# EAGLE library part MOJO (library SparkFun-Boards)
Mojo v3 FPGA Development Board Mechanical footprint with connectors for Mojo FPGA dev board. SparkFun Products: Mojo v3
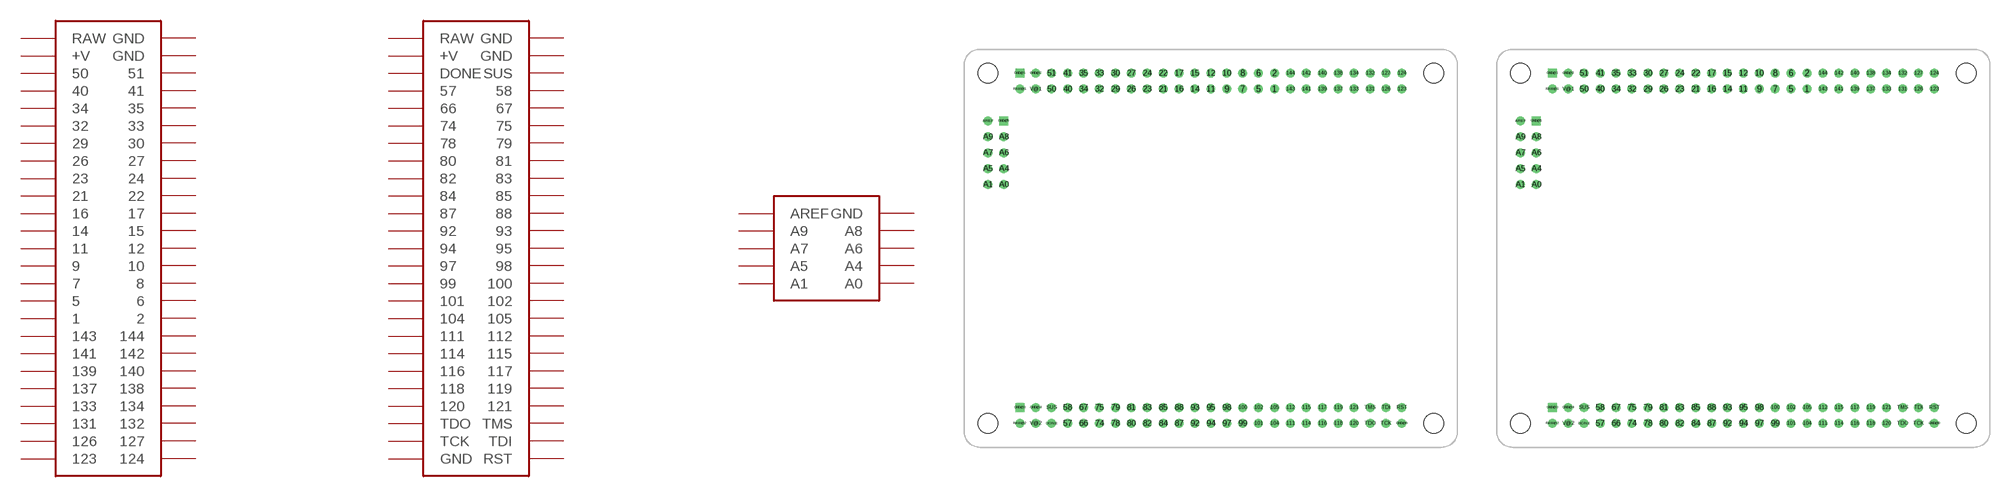
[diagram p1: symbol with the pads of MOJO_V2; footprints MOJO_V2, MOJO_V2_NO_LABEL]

Designator prefix B; gates G$1=MOJO_ANALOG_HEADER G$2=MOJO_HEADER_1 G$3=MOJO_HEADER_2

## MOJOV2  [MOJO_V2]
1  G$2:1
2  G$2:2
5  G$2:5
6  G$2:6
7  G$2:7
8  G$2:8
9  G$2:9
10  G$2:10
11  G$2:11
12  G$2:12
14  G$2:14
15  G$2:15
16  G$2:16
17  G$2:17
21  G$2:21
22  G$2:22
23  G$2:23
24  G$2:24
26  G$2:26
27  G$2:27
29  G$2:29
30  G$2:30
32  G$2:32
33  G$2:33
34  G$2:34
35  G$2:35
40  G$2:40
41  G$2:41
50  G$2:50
51  G$2:51
57  G$3:57
58  G$3:58
66  G$3:66
67  G$3:67
74  G$3:74
75  G$3:75
78  G$3:78
79  G$3:79
80  G$3:80
81  G$3:81
82  G$3:82
83  G$3:83
84  G$3:84
85  G$3:85
87  G$3:87
88  G$3:88
92  G$3:92
93  G$3:93
94  G$3:94
95  G$3:95
97  G$3:97
98  G$3:98
99  G$3:99
100  G$3:100
101  G$3:101
102  G$3:102
104  G$3:104
105  G$3:105
111  G$3:111
112  G$3:112
114  G$3:114
115  G$3:115
116  G$3:116
117  G$3:117
118  G$3:118
119  G$3:119
120  G$3:120
121  G$3:121
123  G$2:123
124  G$2:124
126  G$2:126
127  G$2:127
131  G$2:131
132  G$2:132
133  G$2:133
134  G$2:134
137  G$2:137
138  G$2:138
139  G$2:139
140  G$2:140
141  G$2:141
142  G$2:142
143  G$2:143
144  G$2:144
A0  G$1:A0  in
A1  G$1:A1  in
A4  G$1:A4  in
A5  G$1:A5  in
A6  G$1:A6  in
A7  G$1:A7  in
A8  G$1:A8  in
A9  G$1:A9  in
AREF  G$1:AREF  in
DONE  G$3:DONE
GND@1  G$2:GND  sup
GND@2  G$2:GND  sup
GND@3  G$3:GND  sup
GND@4  G$3:GND  sup
GND@5  G$1:GND  sup
GND@6  G$3:GND  sup
RAW@1  G$2:RAW  sup
RAW@2  G$3:RAW  sup
RST  G$3:RST  in
SUS  G$3:SUS  in
TCK  G$3:TCK  in
TDI  G$3:TDI  in
TDO  G$3:TDO  out
TMS  G$3:TMS  in
V@1  G$2:+V  sup
V@2  G$3:+V  sup

## MOJOV2_NO_LABEL  [MOJO_V2_NO_LABEL]
Pads as for MOJO_V2

## MOJOV3  [MOJO_V3]
Pads as for MOJO_V2

## MOJOV3_NO_LABEL  [MOJO_V3_NO_LABEL]
Pads as for MOJO_V2

## Footprint MOJO_V2 (pad centres in mm)
drill 0.9: 1 49.53,57.15; 2 49.53,59.69; 5 46.99,57.15; 6 46.99,59.69; 7 44.45,57.15; 8 44.45,59.69; 9 41.91,57.15; 10 41.91,59.69; 11 39.37,57.15; 12 39.37,59.69; 14 36.83,57.15; 15 36.83,59.69; 16 34.29,57.15; 17 34.29,59.69; 21 31.75,57.15; 22 31.75,59.69; 23 29.21,57.15; 24 29.21,59.69; 26 26.67,57.15; 27 26.67,59.69; 29 24.13,57.15; 30 24.13,59.69; 32 21.59,57.15; 33 21.59,59.69; 34 19.05,57.15; 35 19.05,59.69; 40 16.51,57.15; 41 16.51,59.69; 50 13.97,57.15; 51 13.97,59.69; 57 16.51,3.81; 58 16.51,6.35; 66 19.05,3.81; 67 19.05,6.35; 74 21.59,3.81; 75 21.59,6.35; 78 24.13,3.81; 79 24.13,6.35; 80 26.67,3.81; 81 26.67,6.35; 82 29.21,3.81; 83 29.21,6.35; 84 31.75,3.81; 85 31.75,6.35; 87 34.29,3.81; 88 34.29,6.35; 92 36.83,3.81; 93 36.83,6.35; 94 39.37,3.81; 95 39.37,6.35; 97 41.91,3.81; 98 41.91,6.35; 99 44.45,3.81; 100 44.45,6.35; 101 46.99,3.81; 102 46.99,6.35; 104 49.53,3.81; 105 49.53,6.35; 111 52.07,3.81; 112 52.07,6.35; 114 54.61,3.81; 115 54.61,6.35; 116 57.15,3.81; 117 57.15,6.35; 118 59.69,3.81; 119 59.69,6.35; 120 62.23,3.81; 121 62.23,6.35; 123 69.85,57.15; 124 69.85,59.69; 126 67.31,57.15; 127 67.31,59.69; 131 64.77,57.15; 132 64.77,59.69; 133 62.23,57.15; 134 62.23,59.69; 137 59.69,57.15; 138 59.69,59.69; 139 57.15,57.15; 140 57.15,59.69; 141 54.61,57.15; 142 54.61,59.69; 143 52.07,57.15; 144 52.07,59.69; A0 6.35,41.91; A1 3.81,41.91; A4 6.35,44.45; A5 3.81,44.45; A6 6.35,46.99; A7 3.81,46.99; A8 6.35,49.53; A9 3.81,49.53; AREF 3.81,52.07; DONE 13.97,3.81; GND@2 11.43,59.69; GND@4 11.43,6.35; GND@6 69.85,3.81; RAW@1 8.89,57.15; RAW@2 8.89,3.81; RST 69.85,6.35; SUS 13.97,6.35; TCK 67.31,3.81; TDI 67.31,6.35; TDO 64.77,3.81; TMS 64.77,6.35; V@1 11.43,57.15; V@2 11.43,3.81
drill 0.9 square: GND@1 8.89,59.69; GND@3 8.89,6.35; GND@5 6.35,52.07
hole 3.2 at 3.81,3.81
hole 3.2 at 3.81,59.69
hole 3.2 at 74.93,59.69
hole 3.2 at 74.93,3.81

## Footprint MOJO_V2_NO_LABEL (pad centres in mm)
drill 0.9: 1 49.53,57.15; 2 49.53,59.69; 5 46.99,57.15; 6 46.99,59.69; 7 44.45,57.15; 8 44.45,59.69; 9 41.91,57.15; 10 41.91,59.69; 11 39.37,57.15; 12 39.37,59.69; 14 36.83,57.15; 15 36.83,59.69; 16 34.29,57.15; 17 34.29,59.69; 21 31.75,57.15; 22 31.75,59.69; 23 29.21,57.15; 24 29.21,59.69; 26 26.67,57.15; 27 26.67,59.69; 29 24.13,57.15; 30 24.13,59.69; 32 21.59,57.15; 33 21.59,59.69; 34 19.05,57.15; 35 19.05,59.69; 40 16.51,57.15; 41 16.51,59.69; 50 13.97,57.15; 51 13.97,59.69; 57 16.51,3.81; 58 16.51,6.35; 66 19.05,3.81; 67 19.05,6.35; 74 21.59,3.81; 75 21.59,6.35; 78 24.13,3.81; 79 24.13,6.35; 80 26.67,3.81; 81 26.67,6.35; 82 29.21,3.81; 83 29.21,6.35; 84 31.75,3.81; 85 31.75,6.35; 87 34.29,3.81; 88 34.29,6.35; 92 36.83,3.81; 93 36.83,6.35; 94 39.37,3.81; 95 39.37,6.35; 97 41.91,3.81; 98 41.91,6.35; 99 44.45,3.81; 100 44.45,6.35; 101 46.99,3.81; 102 46.99,6.35; 104 49.53,3.81; 105 49.53,6.35; 111 52.07,3.81; 112 52.07,6.35; 114 54.61,3.81; 115 54.61,6.35; 116 57.15,3.81; 117 57.15,6.35; 118 59.69,3.81; 119 59.69,6.35; 120 62.23,3.81; 121 62.23,6.35; 123 69.85,57.15; 124 69.85,59.69; 126 67.31,57.15; 127 67.31,59.69; 131 64.77,57.15; 132 64.77,59.69; 133 62.23,57.15; 134 62.23,59.69; 137 59.69,57.15; 138 59.69,59.69; 139 57.15,57.15; 140 57.15,59.69; 141 54.61,57.15; 142 54.61,59.69; 143 52.07,57.15; 144 52.07,59.69; A0 6.35,41.91; A1 3.81,41.91; A4 6.35,44.45; A5 3.81,44.45; A6 6.35,46.99; A7 3.81,46.99; A8 6.35,49.53; A9 3.81,49.53; AREF 3.81,52.07; DONE 13.97,3.81; GND@2 11.43,59.69; GND@4 11.43,6.35; GND@6 69.85,3.81; RAW@1 8.89,57.15; RAW@2 8.89,3.81; RST 69.85,6.35; SUS 13.97,6.35; TCK 67.31,3.81; TDI 67.31,6.35; TDO 64.77,3.81; TMS 64.77,6.35; V@1 11.43,57.15; V@2 11.43,3.81
drill 0.9 square: GND@1 8.89,59.69; GND@3 8.89,6.35; GND@5 6.35,52.07
hole 3.2 at 3.81,3.81
hole 3.2 at 3.81,59.69
hole 3.2 at 74.93,59.69
hole 3.2 at 74.93,3.81

## Footprint MOJO_V3 (pad centres in mm)
drill 1: 1 49.53,57.15; 2 49.53,59.69; 5 46.99,57.15; 6 46.99,59.69; 7 44.45,57.15; 8 44.45,59.69; 9 41.91,57.15; 10 41.91,59.69; 11 39.37,57.15; 12 39.37,59.69; 14 36.83,57.15; 15 36.83,59.69; 16 34.29,57.15; 17 34.29,59.69; 21 31.75,57.15; 22 31.75,59.69; 23 29.21,57.15; 24 29.21,59.69; 26 26.67,57.15; 27 26.67,59.69; 29 24.13,57.15; 30 24.13,59.69; 32 21.59,57.15; 33 21.59,59.69; 34 19.05,57.15; 35 19.05,59.69; 40 16.51,57.15; 41 16.51,59.69; 50 13.97,57.15; 51 13.97,59.69; 57 16.51,3.81; 58 16.51,6.35; 66 19.05,3.81; 67 19.05,6.35; 74 21.59,3.81; 75 21.59,6.35; 78 24.13,3.81; 79 24.13,6.35; 80 26.67,3.81; 81 26.67,6.35; 82 29.21,3.81; 83 29.21,6.35; 84 31.75,3.81; 85 31.75,6.35; 87 34.29,3.81; 88 34.29,6.35; 92 36.83,3.81; 93 36.83,6.35; 94 39.37,3.81; 95 39.37,6.35; 97 41.91,3.81; 98 41.91,6.35; 99 44.45,3.81; 100 44.45,6.35; 101 46.99,3.81; 102 46.99,6.35; 104 49.53,3.81; 105 49.53,6.35; 111 52.07,3.81; 112 52.07,6.35; 114 54.61,3.81; 115 54.61,6.35; 116 57.15,3.81; 117 57.15,6.35; 118 59.69,3.81; 119 59.69,6.35; 120 62.23,3.81; 121 62.23,6.35; 123 69.85,57.15; 124 69.85,59.69; 126 67.31,57.15; 127 67.31,59.69; 131 64.77,57.15; 132 64.77,59.69; 133 62.23,57.15; 134 62.23,59.69; 137 59.69,57.15; 138 59.69,59.69; 139 57.15,57.15; 140 57.15,59.69; 141 54.61,57.15; 142 54.61,59.69; 143 52.07,57.15; 144 52.07,59.69; A0 6.35,41.91; A1 3.81,41.91; A4 6.35,44.45; A5 3.81,44.45; A6 6.35,46.99; A7 3.81,46.99; A8 6.35,49.53; A9 3.81,49.53; AREF 3.81,52.07; DONE 13.97,3.81; GND@2 11.43,59.69; GND@4 11.43,6.35; GND@6 69.85,3.81; RAW@1 8.89,57.15; RAW@2 8.89,3.81; RST 69.85,6.35; SUS 13.97,6.35; TCK 67.31,3.81; TDI 67.31,6.35; TDO 64.77,3.81; TMS 64.77,6.35; V@1 11.43,57.15; V@2 11.43,3.81
drill 1 square: GND@1 8.89,59.69; GND@3 8.89,6.35; GND@5 6.35,52.07
hole 3.2 at 3.81,3.81
hole 3.2 at 3.81,59.69
hole 3.2 at 74.93,59.69
hole 3.2 at 74.93,3.81

## Footprint MOJO_V3_NO_LABEL (pad centres in mm)
drill 1: 1 49.53,57.15; 2 49.53,59.69; 5 46.99,57.15; 6 46.99,59.69; 7 44.45,57.15; 8 44.45,59.69; 9 41.91,57.15; 10 41.91,59.69; 11 39.37,57.15; 12 39.37,59.69; 14 36.83,57.15; 15 36.83,59.69; 16 34.29,57.15; 17 34.29,59.69; 21 31.75,57.15; 22 31.75,59.69; 23 29.21,57.15; 24 29.21,59.69; 26 26.67,57.15; 27 26.67,59.69; 29 24.13,57.15; 30 24.13,59.69; 32 21.59,57.15; 33 21.59,59.69; 34 19.05,57.15; 35 19.05,59.69; 40 16.51,57.15; 41 16.51,59.69; 50 13.97,57.15; 51 13.97,59.69; 57 16.51,3.81; 58 16.51,6.35; 66 19.05,3.81; 67 19.05,6.35; 74 21.59,3.81; 75 21.59,6.35; 78 24.13,3.81; 79 24.13,6.35; 80 26.67,3.81; 81 26.67,6.35; 82 29.21,3.81; 83 29.21,6.35; 84 31.75,3.81; 85 31.75,6.35; 87 34.29,3.81; 88 34.29,6.35; 92 36.83,3.81; 93 36.83,6.35; 94 39.37,3.81; 95 39.37,6.35; 97 41.91,3.81; 98 41.91,6.35; 99 44.45,3.81; 100 44.45,6.35; 101 46.99,3.81; 102 46.99,6.35; 104 49.53,3.81; 105 49.53,6.35; 111 52.07,3.81; 112 52.07,6.35; 114 54.61,3.81; 115 54.61,6.35; 116 57.15,3.81; 117 57.15,6.35; 118 59.69,3.81; 119 59.69,6.35; 120 62.23,3.81; 121 62.23,6.35; 123 69.85,57.15; 124 69.85,59.69; 126 67.31,57.15; 127 67.31,59.69; 131 64.77,57.15; 132 64.77,59.69; 133 62.23,57.15; 134 62.23,59.69; 137 59.69,57.15; 138 59.69,59.69; 139 57.15,57.15; 140 57.15,59.69; 141 54.61,57.15; 142 54.61,59.69; 143 52.07,57.15; 144 52.07,59.69; A0 6.35,41.91; A1 3.81,41.91; A4 6.35,44.45; A5 3.81,44.45; A6 6.35,46.99; A7 3.81,46.99; A8 6.35,49.53; A9 3.81,49.53; AREF 3.81,52.07; DONE 13.97,3.81; GND@2 11.43,59.69; GND@4 11.43,6.35; GND@6 69.85,3.81; RAW@1 8.89,57.15; RAW@2 8.89,3.81; RST 69.85,6.35; SUS 13.97,6.35; TCK 67.31,3.81; TDI 67.31,6.35; TDO 64.77,3.81; TMS 64.77,6.35; V@1 11.43,57.15; V@2 11.43,3.81
drill 1 square: GND@1 8.89,59.69; GND@3 8.89,6.35; GND@5 6.35,52.07
hole 3.2 at 3.81,3.81
hole 3.2 at 3.81,59.69
hole 3.2 at 74.93,59.69
hole 3.2 at 74.93,3.81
